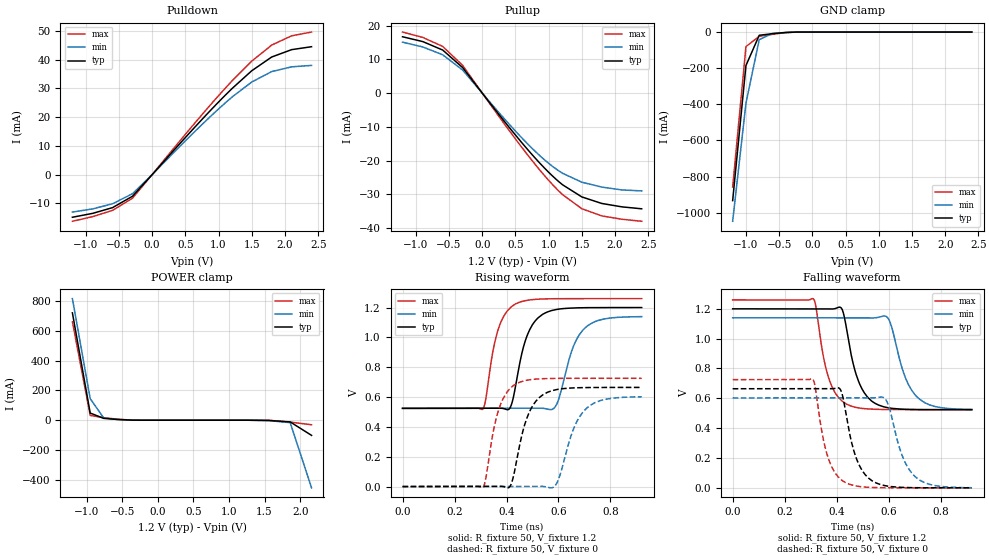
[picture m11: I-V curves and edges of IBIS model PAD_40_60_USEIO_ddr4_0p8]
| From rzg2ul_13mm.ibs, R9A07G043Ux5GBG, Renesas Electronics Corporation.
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[Model] PAD_40_60_USEIO_ddr4_0p8
Model_type I/O
Polarity   Non-Inverting
Vinl = 0.8670
Vinh = 1.0530
Vmeas= 0.960
| Capacitance   typ   min   max
C_comp   2.102e-12   2.013e-12   2.216e-12
[Model Spec]
| Subparameter   typ   min   max
Vmeas   0.960   0.912   1.008
Vinh   1.0530   1.0050   1.1010
Vinl   0.8670   0.8190   0.9150
| Variables   typ   min   max
[GND Clamp Reference]   0   0   0
[POWER Clamp Reference]   1.2   1.14   1.26
[Pulldown Reference]   0   0   0
[Pullup Reference]   1.2   1.14   1.26
[Temperature Range]   25   125   -40
[Voltage Range]   1.2   1.14   1.26
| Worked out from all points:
|   slope of the pulldown table from 0 to 0.18 V, typ, clamps not added: 38.5 ohm
|   slope of the pullup table from 0 to 0.18 V, typ, clamps not added: 39.5 ohm
|   GND clamp passes 1 mA (typ) near -0.30 V on its own axis
|   POWER clamp passes 1 mA (typ) near -0.38 V on its own axis
|   rising waveform, R_fixture 50, V_fixture 1.2: 20-80 % time 59.9ps typ, 68.7ps min, 53.3ps max; typ from 0.524 V to 1.2 V
|   rising waveform, R_fixture 50, V_fixture 0: 20-80 % time 62.9ps typ, 73.3ps min, 55.7ps max; typ from 0 V to 0.665 V
|   falling waveform, R_fixture 50, V_fixture 1.2: 20-80 % time 60.7ps typ, 70.2ps min, 55.4ps max; typ from 1.2 V to 0.524 V
|   falling waveform, R_fixture 50, V_fixture 0: 20-80 % time 60.2ps typ, 68.7ps min, 54.5ps max; typ from 0.664 V to 0 V
[GND Clamp]
| Voltage   I(typ)   I(min)   I(max)
-1.2V     -932.7mA   -1.047A    -857.4mA
-1V       -185.5mA   -394.3mA   -80.64mA
-800mV    -17.89mA   -41.9mA    -23.65mA
-600mV    -9.04mA    -7.411mA   -12.44mA
-400mV    -2.454mA   -2.378mA   -3.185mA
2.4V      0A         0A         0A
[POWER Clamp]
| Voltage   I(typ)   I(min)   I(max)
-1.2V     719.7mA    815.2mA    660.1mA
-950mV    48.1mA     144.6mA    32.07mA
-760mV    12.41mA    14.91mA    17.11mA
-360mV    527.4uA    791.2uA    575.5uA
1.26V     -115.5nA   -12.89uA   -796.6pA
1.56V     -1.53mA    -2.776mA   -549.4uA
1.86V     -11.39mA   -16.33mA   -12.44mA
2.16V     -101.5mA   -453.2mA   -30.39mA
[Pulldown]
| Voltage   I(typ)   I(min)   I(max)
-1.2V     -14.8mA    -13mA      -16.2mA
-895mV    -13.45mA   -11.9mA    -14.59mA
-595mV    -11.45mA   -10.11mA   -12.4mA
-295mV    -7.491mA   -6.611mA   -8.178mA
855mV     21.77mA    19.74mA    23.66mA
1.21V     30.1mA     27.12mA    32.78mA
1.5V      36.14mA    32.23mA    39.49mA
1.8V      40.92mA    35.85mA    45.07mA
2.1V      43.48mA    37.5mA     48.29mA
2.4V      44.5mA     38mA       49.6mA
[Pullup]
| Voltage   I(typ)   I(min)   I(max)
-1.2V     16.7mA     15.1mA     18.1mA
-895mV    15.27mA    13.68mA    16.5mA
-595mV    12.76mA    11.35mA    13.83mA
-295mV    7.559mA    6.831mA    8.212mA
300mV     -7.557mA   -6.876mA   -8.244mA
650mV     -15.96mA   -14.39mA   -17.49mA
955mV     -22.58mA   -20.08mA   -24.87mA
1.21V     -27.19mA   -23.78mA   -30.11mA
1.5V      -30.79mA   -26.42mA   -34.29mA
1.8V      -32.72mA   -27.86mA   -36.41mA
2.1V      -33.72mA   -28.7mA    -37.39mA
2.4V      -34.3mA    -29mA      -38mA
[Ramp]
dV/dt_r   0.4056/5.987e-11   0.3687/6.871e-11   0.4411/5.333e-11
dV/dt_f   0.3986/6.018e-11   0.3611/6.868e-11   0.4352/5.451e-11
R_load= 50
[Rising Waveform]
R_fixture = 50
V_fixture = 1.2
V_fixture_min = 1.14
V_fixture_max = 1.26
| Time   V(typ)   V(min)   V(max)
0s        524mV      524.6mV    524.8mV
309ps     524mV      524.6mV    519mV
360ps     524.4mV    524.6mV    1.005V
408ps     516.8mV    524.6mV    1.187V
487ps     1.044V     524.6mV    1.251V
577ps     1.181V     518.1mV    1.259V
600ps     1.189V     581mV      1.26V
656ps     1.197V     933.6mV    1.26V
700ps     1.199V     1.06V      1.26V
920ps     1.2V       1.139V     1.26V
[Rising Waveform]
R_fixture = 50
V_fixture = 0
V_fixture_min = 0
V_fixture_max = 0
| Time   V(typ)   V(min)   V(max)
0s        95.57nV    4.005uV    16.46nV
309ps     2.574uV    3.821uV    -6.795mV
361ps     483.8uV    3.533uV    462.2mV
409ps     -6.81mV    18.61uV    648.6mV
490ps     507.6mV    63.86uV    716.4mV
579ps     644.6mV    -5.651mV   724.9mV
604ps     653.7mV    67.37mV    725.3mV
658ps     661.5mV    387mV      725.7mV
700ps     663.5mV    511.2mV    725.8mV
920ps     664.6mV    601.8mV    725.8mV
[Falling Waveform]
R_fixture = 50
V_fixture = 1.2
V_fixture_min = 1.14
V_fixture_max = 1.26
| Time   V(typ)   V(min)   V(max)
0s        1.2V       1.14V      1.26V
311ps     1.2V       1.14V      1.266V
363ps     1.2V       1.14V      773.6mV
416ps     1.209V     1.14V      589.5mV
488ps     698mV      1.14V      534.7mV
588ps     540.4mV    1.151V     525.1mV
610ps     533.4mV    1.088V     524.7mV
664ps     526.3mV    740.9mV    524.4mV
704ps     524.6mV    619.5mV    524.4mV
920ps     523.6mV    525.5mV    524.3mV
[Falling Waveform]
R_fixture = 50
V_fixture = 0
V_fixture_min = 0
V_fixture_max = 0
| Time   V(typ)   V(min)   V(max)
0s        664.3mV    602.6mV    725.3mV
308ps     664.3mV    602.6mV    728.9mV
357ps     664mV      602.6mV    262.6mV
410ps     667.6mV    602.6mV    66.82mV
482ps     170.4mV    602.5mV    10.09mV
579ps     17.29mV    606.4mV    769.9uV
600ps     10.38mV    551mV      452.7uV
656ps     2.802mV    199.4mV    117.3uV
700ps     930.6uV    78.51mV    27.93uV
920ps     3.327uV    740.1uV    64.29nV
[Add Submodel]
| Submodel Name Mode
PAD_40_60_0p8_T Non-Driving
